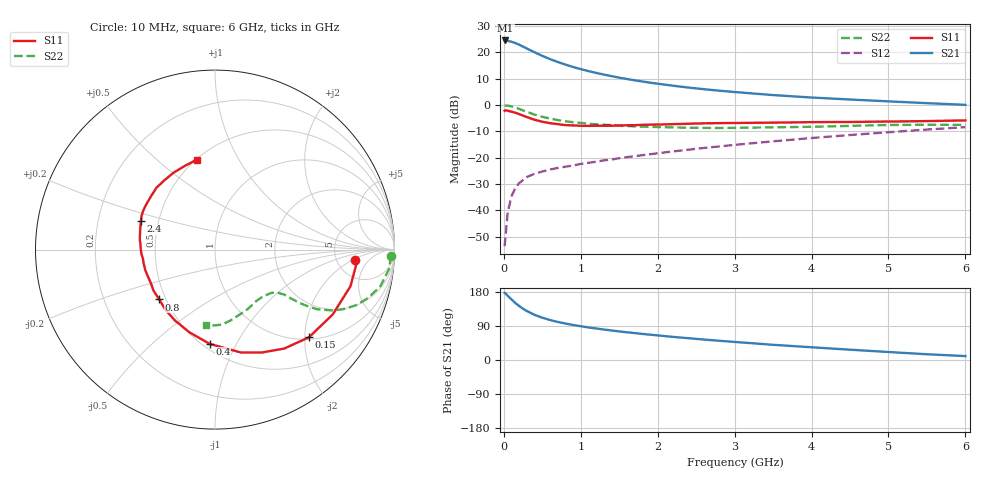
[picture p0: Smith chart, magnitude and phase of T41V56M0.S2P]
! Infineon Technologies  Discrete & RF Semiconductors
! BFR182T
! Si NPN RF Bipolar Junction Transistor in SC75
! VCE = 1.5 V  IC = 6 mA
! Common Emitter S-Parameters:  October  1999
# GHz  S  MA  R  50
!  f  S11  S21  S12  S22
! GHz  MAG  ANG  MAG  ANG  MAG  ANG  MAG  ANG
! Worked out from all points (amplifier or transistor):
!   36 points, 10 MHz to 6 GHz, reference 50 ohm
!   highest |S21| = 24.5 dB at 20 MHz (marker M1)
!   |S21| within 3 dB of that: start of sweep to 295 MHz
!   unconditionally stable (mu >= 1): 1.2 GHz to 4.018 GHz
!   at 250 MHz: K = 0.33, MSG = 25.3 dB, |S12| = -28.4 dB
!   at 1.4 GHz: K = 1.06, MAG = 14.4 dB, |S12| = -20.7 dB
!   at 6 GHz: K = 0.85, MSG = 4.2 dB, |S12| = -8.4 dB
!   lowest NFmin = 1.25 dB at 450 MHz
!   S11 on the Smith chart (normalised r, x): 10 MHz: 7.44, -2.17; 150 MHz: 1.05, -2.10; 400 MHz: 0.54, -0.79; 800 MHz: 0.46, -0.31; 2.4 GHz: 0.40, +0.16; 6 GHz: 0.51, +0.69
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0.01  0.7798 -4.2  16.73 177.2  0.0021 86.6  0.981 -2.0
0.02  0.7942 -4.8  16.85 176.0  0.003 89.9  0.9805 -2.6
0.05  0.7819 -15.1  16.61 169.5  0.0092 81.7  0.9753 -6.5
0.1  0.7491 -28.8  15.9 159.8  0.0187 77.0  0.9438 -12.5
0.15  0.716 -43.0  15.04 150.3  0.0269 69.5  0.894 -17.6
0.2  0.673 -55.0  13.99 142.3  0.0331 66.0  0.8439 -21.6
0.25  0.63 -65.5  12.88 135.2  0.0379 61.2  0.7897 -24.8
0.3  0.5918 -75.8  11.83 129.1  0.0431 58.8  0.7428 -27.2
0.4  0.5261 -93.2  10.05 119.1  0.0499 55.0  0.6588 -30.3
0.5  0.4827 -107.1  8.601 111.7  0.0548 53.3  0.6 -31.5
0.6  0.4539 -119.3  7.458 105.5  0.0598 52.7  0.5549 -32.3
0.7  0.4346 -129.5  6.583 100.5  0.0641 52.7  0.5191 -32.6
0.8  0.4167 -138.2  5.88 96.2  0.0677 52.4  0.4931 -32.8
1.1  0.4029 -159.0  4.419 85.8  0.0803 55.3  0.4439 -33.7
1.4  0.4048 -173.0  3.538 77.9  0.0925 57.2  0.4164 -35.5
1.6  0.4141 179.1  3.124 73.1  0.1027 58.8  0.4013 -36.8
2.2  0.4345 163.3  2.33 61.0  0.132 61.4  0.3778 -43.3
2.4  0.4422 159.1  2.151 57.5  0.1423 61.8  0.3715 -46.0
3.5  0.4641 140.3  1.548 40.1  0.2051 61.2  0.3783 -61.5
4.5  0.4781 126.2  1.276 27.2  0.2704 57.6  0.4026 -76.9
5.5  0.4968 109.2  1.088 15.2  0.3433 52.4  0.423 -90.6
6  0.5112 101.3  1.011 10.3  0.3815 48.8  0.4212 -96.5
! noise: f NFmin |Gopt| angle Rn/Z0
0.45  1.25  0.25  39  0.3
0.9  1.4  0.25  78  0.23
1.8  1.95  0.21  151  0.2
